PROGRAM MAIN
VAR
	mcPowerMaster: MC_Power;
	mcPowerSlave: MC_Power;
	fbSmoothCam: FB_SmoothCam;
	TESTMOVE:MC_MOVEVELOCITY;
	TEST_START: BOOL;
END_VAR

mcPowerMaster(
	Axis:= Master, 
	Enable:=TRUE , 
	Enable_Positive:=TRUE , 
	Enable_Negative:=TRUE , 
	Override:=100 , 
	BufferMode:= , 
	Options:= , 
	Status=> , 
	Busy=> , 
	Active=> , 
	Error=> , 
	ErrorID=> );
	
mcPowerSlave(
	Axis:= Slave, 
	Enable:=TRUE , 
	Enable_Positive:=TRUE , 
	Enable_Negative:=TRUE , 
	Override:=100 , 
	BufferMode:= , 
	Options:= , 
	Status=> , 
	Busy=> , 
	Active=> , 
	Error=> , 
	ErrorID=> );
TESTMOVE(                                 //启动主轴运转 
	Axis:= MASTER, 
	Execute:= TEST_START, 
	Velocity:=10 ,  );
fbSmoothCam(
	Execute:=fbSmoothCam.Execute ,        //启动平滑凸轮耦合
	CamTableID:=3 , 
	CamTableIDAcc:=4 , 
	Done=> , 
	Busy=> , 
	Error=> , 
	ErrorID=> , 
	Master:=Master , 
	Slave:=Slave );

END_PROGRAM
